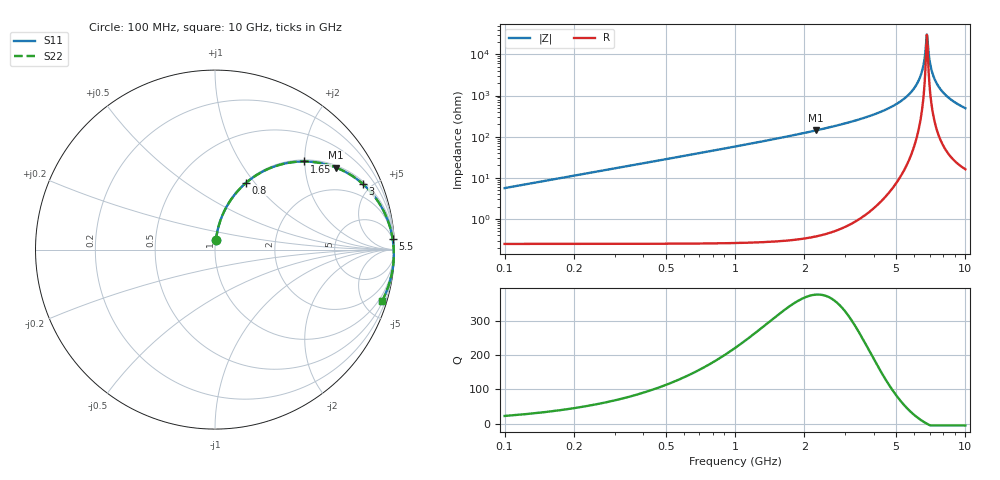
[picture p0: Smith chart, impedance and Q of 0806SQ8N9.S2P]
! Coilcraft 0806SQ-8N9 Air Core Inductor
! 06 March 2008
# MHZ S MA R 50
!Freq  MagS11  AngS11  MagS21  AngS21  MagS12  AngS12  MagS22  AngS22
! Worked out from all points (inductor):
!   397 points, 100 MHz to 10 GHz, reference 50 ohm
!   read as one part in series: L = 8.96 nH near 125 MHz
!   highest Q = 377 at 2.25 GHz (marker M1), where L = 10.1 nH
!   self-resonance near 6.8 GHz
!   S11 on the Smith chart (normalised r, x): 100 MHz: 1.01, +0.11; 800 MHz: 1.01, +0.91; 1.65 GHz: 1.04, +1.99; 3 GHz: 1.14, +4.42; 5.5 GHz: 5, +33; 10 GHz: 0.59, -6.65
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100  0.05568 84.2  0.996 -3.2  0.996 -3.2  0.05569 84.2
200  0.1108 82.3  0.9914 -6.5  0.9914 -6.5  0.1108 82.3
350  0.1919 78.0  0.979 -11.2  0.979 -11.2  0.1919 78.0
800  0.4118 64.9  0.9089 -24.7  0.9089 -24.7  0.4118 64.9
1650  0.6987 44.6  0.7133 -45.2  0.7133 -45.2  0.6988 44.6
1750  0.7222 42.7  0.6896 -47.2  0.6896 -47.2  0.7222 42.7
2250  0.8151 34.1  0.5771 -55.8  0.5771 -55.8  0.8152 34.1
3000  0.9005 24.0  0.4321 -65.8  0.4321 -65.8  0.9006 24.0
3400  0.9292 19.7  0.3661 -70.1  0.3661 -70.1  0.9293 19.7
5050  0.9857 6.3  0.1561 -83.0  0.1561 -83.0  0.9858 6.3
5500  0.9915 3.4  0.1112 -85.4  0.1112 -85.4  0.9916 3.4
6325  0.9964 -1.2  0.03831 -87.0  0.03831 -87.0  0.9965 -1.2
6550  0.9968 -2.4  0.02029 -83.9  0.02029 -83.9  0.9968 -2.4
6700  0.9968 -3.2  0.008906 -72.6  0.008906 -72.6  0.9969 -3.2
6800  0.9968 -3.7  0.003273 -15.6  0.003273 -15.6  0.9968 -3.7
6825  0.9967 -3.8  0.003446 16.9  0.003446 16.9  0.9968 -3.8
6900  0.9966 -4.1  0.007611 60.3  0.007611 60.3  0.9967 -4.1
6975  0.9965 -4.5  0.01289 70.4  0.01289 70.4  0.9966 -4.5
7225  0.9959 -5.7  0.0308 77.7  0.0308 77.7  0.996 -5.7
7675  0.9941 -7.7  0.06176 78.6  0.06176 78.6  0.9942 -7.7
8350  0.9898 -10.6  0.1048 76.8  0.1048 76.8  0.9899 -10.6
10000  0.9743 -17.0  0.1956 71.2  0.1956 71.2  0.9744 -17.0
